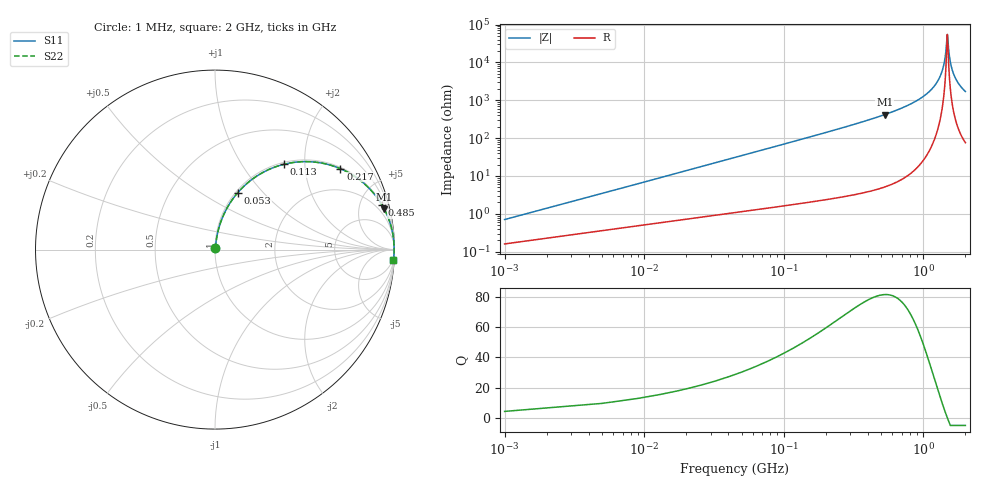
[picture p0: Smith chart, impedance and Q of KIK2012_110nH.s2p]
!version-2
!date-01.2022
!Series
# MHz S RI R 50
!Freq ReS11 ImS11 ReS21 ImS21 ReS12 ImS12 ReS22 ImS22
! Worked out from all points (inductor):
!   501 points, 1 MHz to 2 GHz, reference 50 ohm
!   read as one part in series: L = 110 nH near 9 MHz
!   highest Q = 81.5 at 529 MHz (marker M1), where L = 126 nH
!   self-resonance near 1.485 GHz
!   S11 on the Smith chart (normalised r, x): 1 MHz: 1.00, +0.01; 53 MHz: 1.02, +0.73; 113 MHz: 1.03, +1.57; 217 MHz: 1.05, +3.06; 485 MHz: 1.09, +7.50; 2 GHz: 3, -34
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1  0.00166 0.00689  0.9983 -0.00689  0.9983 -0.00689  0.00166 0.00689
13  0.0137 0.0881  0.9863 -0.0881  0.9863 -0.0881  0.0137 0.0881
17  0.02 0.1144  0.98 -0.1144  0.98 -0.1144  0.02 0.1144
33  0.0574 0.2131  0.9426 -0.2131  0.9426 -0.2131  0.0574 0.2131
53  0.1264 0.3167  0.8736 -0.3167  0.8736 -0.3167  0.1264 0.3167
113  0.3842 0.4755  0.6158 -0.4755  0.6158 -0.4755  0.3842 0.4755
217  0.6985 0.4509  0.3015 -0.4509  0.3015 -0.4509  0.6985 0.4509
337  0.8544 0.346  0.1456 -0.346  0.1456 -0.346  0.8544 0.346
485  0.931 0.2473  0.069 -0.2473  0.069 -0.2473  0.931 0.2473
529  0.9436 0.2247  0.0564 -0.2247  0.0564 -0.2247  0.9436 0.2247
669  0.9691 0.1667  0.0309 -0.1667  0.0309 -0.1667  0.9691 0.1667
1001  0.9922 0.0781  0.00778 -0.0781  0.00778 -0.0781  0.9922 0.0781
1205  0.9967 0.0408  0.0033 -0.0408  0.0033 -0.0408  0.9967 0.0408
1337  0.9979 0.0205  0.00211 -0.0205  0.00211 -0.0205  0.9979 0.0205
1425  0.9982 0.00806  0.00183 -0.00806  0.00183 -0.00806  0.9982 0.00806
1485  0.9982 5.34e-05  0.00183 -5.34e-05  0.00183 -5.34e-05  0.9982 5.34e-05
1493  0.9982 -0.000989  0.00184 0.000989  0.00184 0.000989  0.9982 -0.000989
1525  0.9981 -0.0051  0.0019 0.0051  0.0019 0.0051  0.9981 -0.0051
1557  0.998 -0.00914  0.002 0.00914  0.002 0.00914  0.998 -0.00914
1669  0.9974 -0.0226  0.00257 0.0226  0.00257 0.0226  0.9974 -0.0226
1809  0.9962 -0.0384  0.00376 0.0384  0.00376 0.0384  0.9962 -0.0384
2000  0.994 -0.0583  0.00604 0.0583  0.00604 0.0583  0.994 -0.0583
